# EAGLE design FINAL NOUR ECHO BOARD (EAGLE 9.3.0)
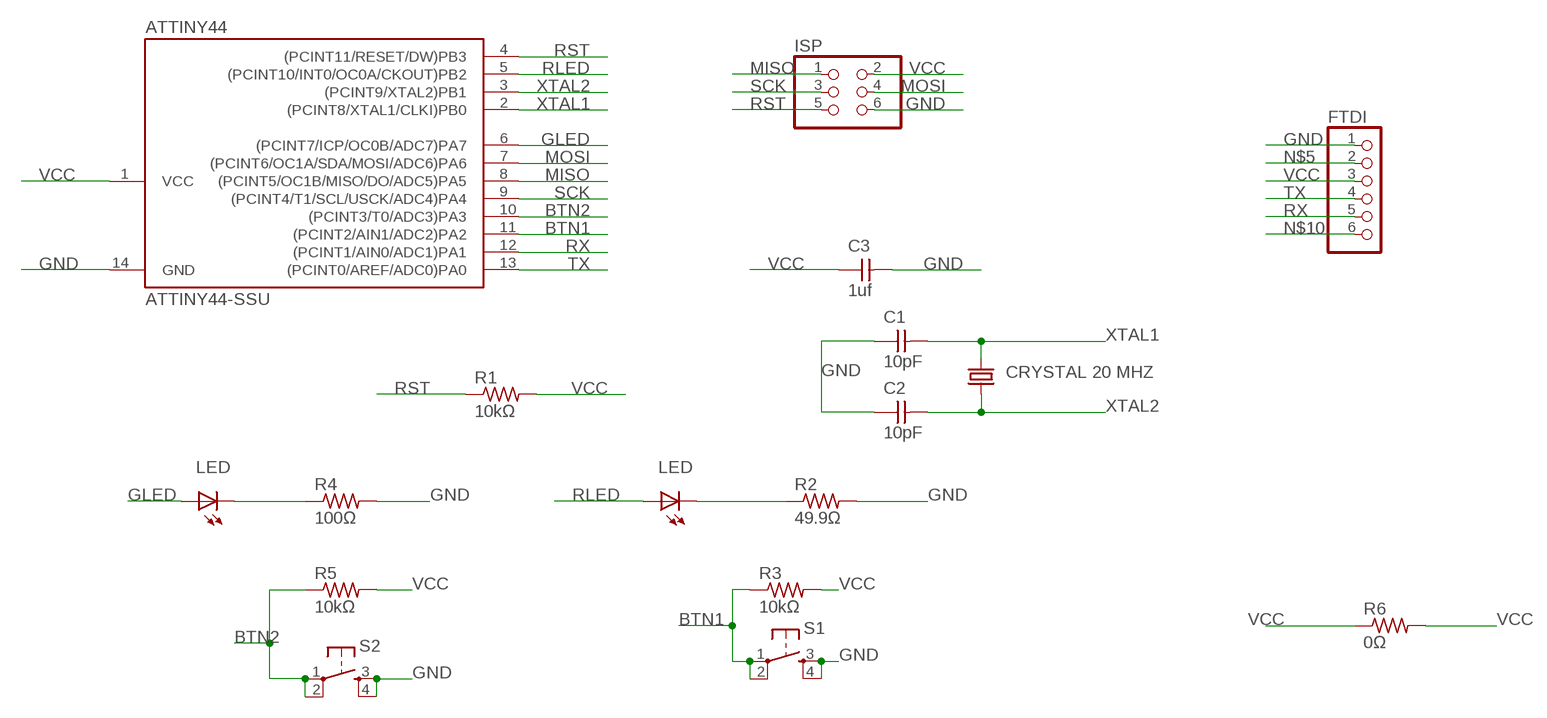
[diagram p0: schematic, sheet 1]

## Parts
ATTINY44  ATTINY44-SSU  [SOIC14]
C1  10pF  CAP-UNPOLARIZEDFAB  [C1206FAB]
C2  10pF  CAP-UNPOLARIZEDFAB  [C1206FAB]
C3  1uf  CAP-UNPOLARIZEDFAB  [C1206FAB]
FTDI  PINHD-1X6  [1X06]
ISP  PINHD-2X3-SMD  [2X03SMD]
R1  10kΩ  RES-US1206FAB  [R1206FAB]
R2  49.9Ω  RES-US1206FAB  [R1206FAB]
R3  10kΩ  RES-US1206FAB  [R1206FAB]
R4  100Ω  RES-US1206FAB  [R1206FAB]
R5  10kΩ  RES-US1206FAB  [R1206FAB]
R6  0Ω  RES-US1206FAB  [R1206FAB]
S1  6MM_SWITCH6MM_SWITCH  [6MM_SWITCH]
S2  6MM_SWITCH6MM_SWITCH  [6MM_SWITCH]
U$1  CRYSTAL 20 MHZ  CRYSTAL  [2-SMD-5X3MM]
U$3  LED  [LED1206]
U$4  LED  [LED1206]

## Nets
BTN1: ATTINY44.11((PCINT2/AIN1/ADC2)PA2) R3.1 S1.1(P) S1.2(P1)
BTN2: ATTINY44.10((PCINT3/T0/ADC3)PA3) R5.1 S2.1(P) S2.2(P1)
GLED: ATTINY44.6((PCINT7/ICP/OC0B/ADC7)PA7) U$4.1(A)
GND: ATTINY44.14(GND) C1.1 C2.1 C3.2 FTDI.1 ISP.6 R2.2 R4.2 S1.3(S) S1.4(S1) S2.3(S) S2.4(S1)
MISO: ATTINY44.8((PCINT5/OC1B/MISO/DO/ADC5)PA5) ISP.1
MOSI: ATTINY44.7((PCINT6/OC1A/SDA/MOSI/ADC6)PA6) ISP.4
N$1: R2.1 U$3.2(C)
N$4: R4.1 U$4.2(C)
N$5: FTDI.2
N$10: FTDI.6
RLED: ATTINY44.5((PCINT10/INT0/OC0A/CKOUT)PB2) U$3.1(A)
RST: ATTINY44.4((PCINT11/RESET/DW)PB3) ISP.5 R1.1
RX: ATTINY44.12((PCINT1/AIN0/ADC1)PA1) FTDI.5
SCK: ATTINY44.9((PCINT4/T1/SCL/USCK/ADC4)PA4) ISP.3
TX: ATTINY44.13((PCINT0/AREF/ADC0)PA0) FTDI.4
VCC: ATTINY44.1(VCC) C3.1 FTDI.3 ISP.2 R1.2 R3.2 R5.2 R6.1 R6.2
XTAL1: ATTINY44.2((PCINT8/XTAL1/CLKI)PB0) C1.2 U$1.P$2
XTAL2: ATTINY44.3((PCINT9/XTAL2)PB1) C2.2 U$1.P$1

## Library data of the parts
ATTINY44 = fab:ATTINY44
C1-C3 = fab:CAP-UNPOLARIZED
FTDI = pinhead:PINHD-1X6: PIN HEADER
ISP = fab:PINHD-2X3-SMD: PIN HEADER
R1-R6 = fab:RES-US: Resistor (US Symbol)
S1 S2 = fab:6MM_SWITCH: OMRON SWITCH
U$1 = fab:CRYSTAL
U$3 U$4 = fab:LED: LED

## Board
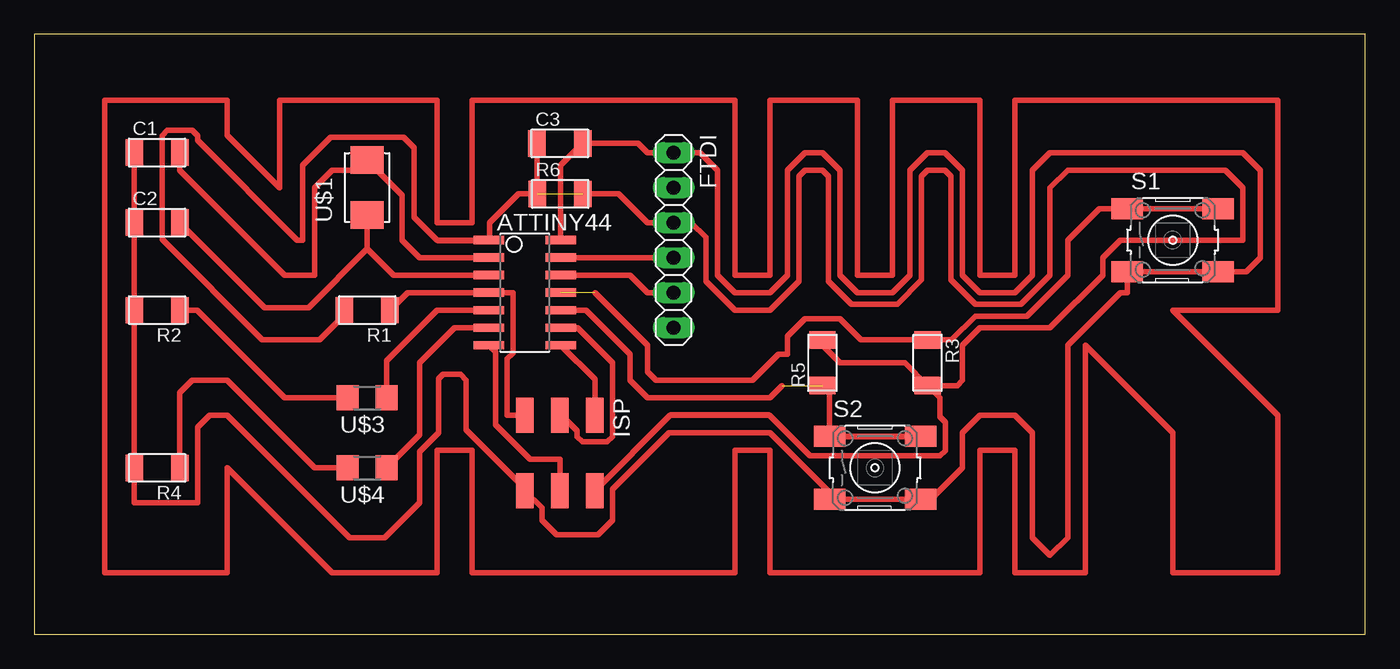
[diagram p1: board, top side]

Size 96.5 x 43.48 mm. Coordinates in mm from the lower left corner, seen from the top.
Outline: 0,0 96.5,0 96.5,43.48 0,43.48 0,0
Copper layers (1*16): Top 0.035mm / dielectric 1.5mm / Bottom 0.035mm
Design rules "default *": minimum track width 16mil, minimum drill 0.35mm, track to track 17mil, track to pad 17mil, pad to pad 17mil, via to via 17mil, smd to smd 17mil, copper to edge 17mil, drill to drill 17mil, minimum pad ring 10mil, minimum via ring 8mil, stop-mask expansion 4mil, vias tented up to drill 0mil, thermal gap 10mil

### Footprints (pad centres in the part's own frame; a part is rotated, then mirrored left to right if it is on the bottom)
SOIC14 = smd 0.61 x 2.21: 1 -3.81,-2.603; 2 -2.54,-2.603; 3 -1.27,-2.603; 4 0,-2.603; 5 1.27,-2.603; 6 2.54,-2.603; 7 3.81,-2.603; 8 3.81,2.603; 9 2.54,2.603; 10 1.27,2.603; 11 0,2.603; 12 -1.27,2.603; 13 -2.54,2.603; 14 -3.81,2.603
C1206FAB = smd 1.27 x 1.905: 1 -1.651,0; 2 1.651,0
1X06 = drill 1.016 long: 1 -6.35,0; 2 -3.81,0; 3 -1.27,0; 4 1.27,0; 5 3.81,0; 6 6.35,0
2X03SMD = smd 2.54 x 1.27: 1 -2.54,2.54; 2 2.92,2.54; 3 -2.54,0; 4 2.92,0; 5 -2.54,-2.54; 6 2.92,-2.54
R1206FAB = smd 1.27 x 1.905: 1 -1.651,0; 2 1.651,0
6MM_SWITCH = smd 2.286 x 1.524: 1 -3.302,2.286; 2 3.302,2.286; 3 -3.302,-2.286; 4 3.302,-2.286
2-SMD-5X3MM = smd 2 x 2.4: P$1 -2,0; P$2 2,0
LED1206 = smd 1.6 x 1.803: 1 -1.422,0; 2 1.422,0

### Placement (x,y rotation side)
ATTINY44  35.56,24.77 270 top
C1  8.89,34.92 0 top
C2  8.89,29.84 0 top
C3  38.1,35.59 0 top
FTDI  46.36,28.58 270 top
ISP  38.1,13.33 270 top
R1  24.13,23.5 180 top
R2  8.89,23.5 180 top
R3  64.77,19.69 270 top
R4  8.89,12.06 180 top
R5  57.15,19.69 90 top
R6  38.13,31.93 0 top
S1  82.55,28.58 0 top
S2  60.96,12.06 0 top
U$1  24.13,32.39 90 top
U$3  24.13,17.14 180 top
U$4  24.13,12.06 180 top

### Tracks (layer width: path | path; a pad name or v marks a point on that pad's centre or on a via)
BTN1  (1 unrouted)
  Top 0.406: S1.2 S1.1 77.22,30.86 74.93,28.58 74.93,26.03 71.96,23.06 68.23,23.06 66.51,21.34 R3.1 | 64.39,20.95 R3.1 | 40.64,24.77 44.45,20.95 44.45,19.05 45.08,18.42 52.07,18.42 53.97,20.32 54.61,20.32 54.61,21.59 55.88,22.86 58.42,22.86 59.94,21.34 R3.1
BTN2  (1 unrouted)
  Top 0.406: 57.66,17.53 S2.1 | 54.23,18.03 53.34,17.14 44.45,17.14 43.18,18.42 43.18,20.32 40,23.5 ATTINY44.10
  Top 0.432: S2.1 S2.2 | R5.1 57.66,17.53
GLED
  Top 0.406: U$4.1 27.94,14.45 27.94,19.69 30.48,22.22 ATTINY44.6
GND
  Top 0.406: C1.1 C2.1 R2.2 R4.2 7.24,9.53 11.82,9.53 11.82,15 12.7,15.88 13.97,15.88 22.86,6.98 25.4,6.98 27.94,9.53 27.94,13.23 29.31,14.61 29.31,18.52 29.64,18.85 30.89,18.85 31.32,18.42 31.32,14.84 35.56,10.6 ISP.6 36.82,9.16 36.82,8.27 37.86,7.23 40.88,7.23 41.91,8.25 41.91,10.5 46.02,14.61 53.34,14.61 58.17,9.78 | S2.3 58.17,9.78 | 58.17,9.78 S2.4 65.02,9.78 67.31,12.06 67.31,14.61 68.58,15.88 71.12,15.88 72.39,14.61 72.39,6.98 73.66,5.71 74.93,6.98 74.93,20.95 78.74,24.77 79.25,24.77 S1.3 S1.4 | 86.11,26.03 S1.4 | S1.4 87.88,26.29 88.9,27.3 88.9,33.66 87.63,34.92 73.66,34.92 72.39,33.66 72.39,26.03 71.12,24.77 68.58,24.77 67.31,26.03 67.31,33.66 66.04,34.92 64.77,34.92 63.5,33.66 63.5,26.03 62.23,24.77 59.69,24.77 58.42,26.03 58.42,33.66 57.15,34.92 55.88,34.92 54.61,33.66 54.61,26.03 53.34,24.77 50.8,24.77 49.53,26.03 49.53,33.66 48.26,34.92 FTDI.1 44.45,34.92 43.79,35.58 C3.2 38.16,34 ATTINY44.14
  Top 0.432: 57.4,9.53 S2.3
GROUND
  Top 0.406: 13.97,4.45 5.08,4.45 5.08,38.73 13.97,38.73 13.97,36.19 17.78,32.39 17.78,38.73 29.21,38.73 29.21,29.84 31.75,29.84 31.75,38.73 50.8,38.73 50.8,26.03 53.34,26.03 53.34,38.73 59.69,38.73 59.69,26.03 62.23,26.03 62.23,38.73 68.58,38.73 68.58,26.03 71.12,26.03 71.12,38.73 90.17,38.73 90.17,23.5 82.55,23.5 90.17,15.88 90.17,4.45 82.55,4.45 82.55,14.61 76.2,20.95 76.2,4.45 71.12,4.45 71.12,13.33 68.58,13.33 68.58,4.45 53.34,4.45 53.34,13.33 50.8,13.33 50.8,4.45 31.75,4.45 31.75,13.33 29.21,13.33 29.21,4.45 21.59,4.45 13.97,12.06 13.97,4.45
MISO
  Top 0.406: ATTINY44.8 40.64,18.48 ISP.1
MOSI
  Top 0.406: ISP.4 38.1,12.69 35.93,12.69 33.43,15.19 33.43,20.48
  Top 0.432: ATTINY44.7 33.43,20.48
N$1
  Top 0.406: R2.1 11.81,23.5 18.16,17.14 U$3.2
N$4
  Top 0.406: R4.1 10.54,17.53 11.43,18.42 13.97,18.42 20.32,12.06 U$4.2
RLED
  Top 0.406: U$3.1 25.55,19.84 29.21,23.5 ATTINY44.5
RST
  Top 0.406: R1.1 27.05,24.77 ATTINY44.4 34.71,24.77 34.71,24.07 34.71,23.5 34.71,20.38 34.29,19.96 34.29,15.88 ISP.5
RX
  Top 0.406: FTDI.5 44.45,24.77 43.18,26.03 ATTINY44.12
SCK
  Top 0.406: 38.16,15.94 39.36,14.75 39.36,14.34 39.74,13.96 41.54,13.96 41.92,14.34 41.92,19.67 39.37,22.22 ATTINY44.9
  Top 0.432: 38.16,15.94 ISP.3
TX
  Top 0.406: ATTINY44.13 FTDI.4
VCC  (1 unrouted)
  Top 0.406: R1.2 22.48,23.16 20.68,21.36 16.52,21.36 9.26,28.62 9.26,36.15 9.64,36.53 11.44,36.53 11.82,36.15 11.82,35.8 19.05,28.58 19.46,28.58 19.46,34.01 21.48,36.03 26.78,36.03 27.53,35.28 27.53,30.25 29.21,28.58 | 53.31,15.88 56.25,12.94 65.67,12.94 66.05,13.32 66.05,15.38 65.67,15.76 65.67,17.13 R3.2 | 46.1,15.88 ISP.2 | 33.4,28.58 33.02,28.58 | 33.02,28.58 ATTINY44.1 | R3.2 66.93,18.03 67.31,18.42 67.31,20.95 68.58,22.22 73.66,22.22 77.47,26.03 77.47,27.3 78.74,28.58 87.63,28.58 87.63,32.39 86.36,33.66 74.93,33.66 73.66,32.39 73.66,26.03 71.55,23.93 68.23,23.93 66.47,25.69 66.47,33.22 66.04,33.66 64.77,33.66 64.34,33.22 64.34,25.69 62.58,23.93 59.26,23.93 57.58,25.6 57.58,33.22 57.15,33.66 55.88,33.66 55.45,33.22 55.45,25.6 53.34,23.5 50.8,23.5 48.69,25.6 48.69,28.78 47.62,29.84 FTDI.3 | R3.2 63.12,19.69 58.42,19.69 57.15,20.95 R5.2 | 46.99,29.84 FTDI.3 | 35.97,35.56 C3.1 36.45,31.95 R6.1 35.1,31.93 33.02,29.84 33.02,28.58 | R6.2 42.37,31.93 44.45,29.84 FTDI.3
  Top 0.432: 29.21,28.58 ATTINY44.1 33.02,28.64 | 53.31,15.88 46.1,15.88
XTAL1
  Top 0.406: C1.2 10.54,33.66 18.16,26.03 20.32,26.03 20.32,32.39 21.59,33.66 23.4,33.66 | 24.86,33.66 26.67,31.84 26.67,28.58 27.94,27.3 ATTINY44.2
  Top 0.432: 23.4,33.66 U$1.P$2 24.86,33.66
XTAL2
  Top 0.406: C2.2 16.7,23.69 19.88,23.69 24.13,27.94 | 24.13,27.94 U$1.P$1 | ATTINY44.3 26.03,26.03 24.13,27.94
